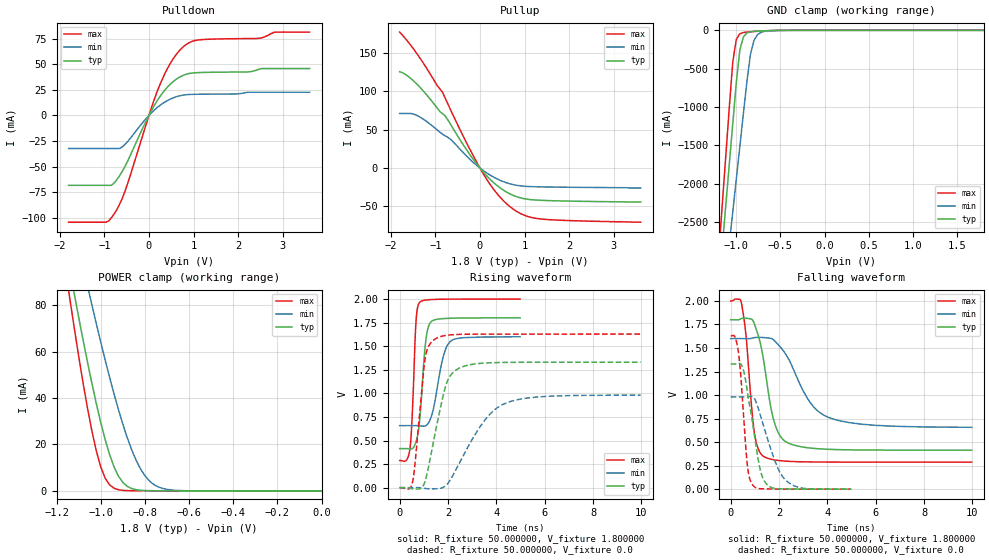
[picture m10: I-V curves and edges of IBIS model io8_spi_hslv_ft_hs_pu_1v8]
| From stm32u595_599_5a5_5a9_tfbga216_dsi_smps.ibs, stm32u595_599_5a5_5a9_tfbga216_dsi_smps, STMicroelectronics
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|   Model io8_spi_hslv_ft_hs_pu_1v8
[Model]  io8_spi_hslv_ft_hs_pu_1v8
Model_type I/O
Polarity   Non-Inverting
Enable   Active-Low
Vinl =   0.540000V
Vinh =   1.260000V
Vmeas =  0.900000V
Cref =   50.000000pF
Rref =   100.000000M
Vref =   0.0V
C_comp   3.338700pF   3.332500pF   3.379000pF
[Temperature Range]   25.000000   0.140000k   -40.000000
[Pullup Reference]   1.800000V   1.600000V   2.000000V
[Pulldown Reference]   0.0V   0.0V   0.0V
[POWER Clamp Reference]   1.800000V   1.600000V   2.000000V
[GND Clamp Reference]   0.0V   0.0V   0.0V
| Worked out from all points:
|   slope of the pulldown table from 0 to 0.27 V, typ, clamps not added: 13.6 ohm
|   slope of the pullup table from 0 to 0.27 V, typ, clamps not added: 15.9 ohm
|   GND clamp passes 1 mA (typ) near -0.51 V on its own axis
|   POWER clamp passes 1 mA (typ) near -0.86 V on its own axis
|   rising waveform, R_fixture 50.000000, V_fixture 1.800000: 20-80 % time 248ps typ, 425ps min, 162ps max; typ from 0.415 V to 1.8 V
|   rising waveform, R_fixture 50.000000, V_fixture 0.0: 20-80 % time 658ps typ, 1.41ns min, 354ps max; typ from 0 V to 1.33 V
|   falling waveform, R_fixture 50.000000, V_fixture 1.800000: 20-80 % time 579ps typ, 1.21ns min, 341ps max; typ from 1.8 V to 0.415 V
|   falling waveform, R_fixture 50.000000, V_fixture 0.0: 20-80 % time 499ps typ, 774ps min, 276ps max; typ from 1.33 V to 0 V
[Pulldown]
|Voltage   I(typ)   I(min)   I(max)
-1.8V     -68.38mA   -32.32mA   -104.4mA
-960mV    -68.38mA   -32.32mA   -104.4mA
-780mV    -66.07mA   -32.32mA   -96.42mA
-540mV    -50.22mA   -28.51mA   -74.66mA
0V        0A         0A         0A
240mV     18.04mA    9.599mA    29.41mA
480mV     30.68mA    16.02mA    50.95mA
780mV     39.47mA    19.98mA    67.56mA
1.14V     41.98mA    20.78mA    74.01mA
2.46V     45.09mA    22.68mA    75.44mA
2.82V     45.89mA    22.68mA    81.56mA
3.6V      45.89mA    22.68mA    81.56mA
[Pullup]
|Voltage   I(typ)   I(min)   I(max)
-1.8V     125.5mA    71.12mA    177.1mA
-1.5V     114.2mA    70.55mA    156mA
-1.32V    103.6mA    65.58mA    141.1mA
-840mV    70.93mA    44.11mA    98.76mA
-660mV    57.08mA    37.46mA    76.03mA
-360mV    29.01mA    19.22mA    39.75mA
60mV      -4.209mA   -2.643mA   -6.075mA
360mV     -21.65mA   -13.44mA   -31.67mA
660mV     -33.29mA   -20.31mA   -49.69mA
960mV     -39.54mA   -23.52mA   -60.64mA
1.32V     -41.88mA   -24.45mA   -66.02mA
3.6V      -44.3mA    -26mA      -70.5mA
[GND_clamp]
|Voltage   I(typ)   I(min)   I(max)
-1.8V     -9.908A    -9.683A    -9.994A
-1.2V     -3.383A    -4.084A    -2.934A
-1.16V    -2.841A    -3.655A    -2.294A
-1.12V    -2.299A    -3.226A    -1.656A
-1.04V    -1.218A    -2.369A    -414.2mA
-1V       -684.7mA   -1.941A    -119.2mA
-960mV    -257.2mA   -1.514A    -45.66mA
-920mV    -87.03mA   -1.089A    -28.93mA
-840mV    -19.35mA   -312.8mA   -18.96mA
-800mV    -13.55mA   -132.4mA   -15.49mA
-720mV    -8.042mA   -25.66mA   -9.49mA
1.8V      0A         13.64nA    0A
[POWER_clamp]
|Voltage   I(typ)   I(min)   I(max)
-1.8V     470.9mA    433.7mA    554.6mA
-1.14V    95.28mA    122.7mA    82.88mA
-1.12V    85mA       114mA      70.34mA
-1.06V    55.55mA    88.43mA    35.73mA
-1.04V    46.38mA    80.17mA    25.83mA
-1V       29.54mA    64.14mA    10.37mA
-940mV    10.43mA    41.88mA    1.177mA
-900mV    3.66mA     28.79mA    250.5uA
-840mV    527.2uA    13.26mA    95.94uA
-800mV    154uA      6.55mA     88.41uA
-740mV    59.83uA    1.741mA    70.38uA
0V        0A         18.18nA    0A
[Ramp]
| variable   typ   min   max
dV/dt_r  0.79756/0.65629n   0.58781/1.41201n   0.97651/0.35346n
dV/dt_f  0.83129/0.57799n   0.56431/1.20386n   1.02742/0.34085n
R_load = 50.000000
[Rising Waveform]
R_fixture= 50.000000
V_fixture= 1.800000
V_fixture_min= 1.600000
V_fixture_max= 2.000000
|time   V(typ)   V(min)   V(max)
0s        414.5mV    657.6mV    287.8mV
440.4ps   408.4mV    657.7mV    442.3mV
530.5ps   414.7mV    657.8mV    823.4mV
670.7ps   480.5mV    657.7mV    1.731V
820.8ps   695.4mV    656mV      1.961V
1.081ns   1.554V     657.1mV    1.988V
1.301ns   1.758V     748.1mV    1.994V
1.802ns   1.792V     1.385V     1.998V
2.082ns   1.795V     1.547V     1.998V
4.985ns   1.8V       1.6V       1.999V
[Rising Waveform]
R_fixture= 50.000000
V_fixture= 0.0
V_fixture_min= 0.0
V_fixture_max= 0.0
|time   V(typ)   V(min)   V(max)
0s        405.1uV    502.6uV    493.5uV
520.5ps   -10.97mV   536.3uV    44.51mV
620.6ps   -13.8mV    627.3uV    214.3mV
1.061ns   74.82mV    -7.697mV   1.383V
1.481ns   593.5mV    -11.54mV   1.578V
1.982ns   1.134V     40.72mV    1.616V
2.683ns   1.289V     363.7mV    1.626V
3.724ns   1.323V     776.7mV    1.628V
4.565ns   1.328V     912.1mV    1.628V
9.97ns    1.33V      980.7mV    1.628V
[Falling Waveform]
R_fixture= 50.000000
V_fixture= 1.800000
V_fixture_min= 1.600000
V_fixture_max= 2.000000
|time   V(typ)   V(min)   V(max)
0s        1.8V       1.6V       1.999V
440.4ps   1.813V     1.6V       1.985V
640.6ps   1.817V     1.599V     1.615V
981ps     1.756V     1.61V      601.7mV
1.361ns   1.371V     1.611V     348.3mV
1.842ns   682.3mV    1.57V      309.9mV
2.422ns   485.8mV    1.37V      295.8mV
3.283ns   437.4mV    923.5mV    289.8mV
4.104ns   423.4mV    757.7mV    288.3mV
9.97ns    414.5mV    657.6mV    287.8mV
[Falling Waveform]
R_fixture= 50.000000
V_fixture= 0.0
V_fixture_min= 0.0
V_fixture_max= 0.0
|time   V(typ)   V(min)   V(max)
0s        1.33V      980.7mV    1.628V
170.2ps   1.33V      980.7mV    1.621V
310.3ps   1.333V     980.8mV    1.474V
510.5ps   1.282V     980.6mV    866.6mV
690.7ps   1.036V     982.1mV    253.9mV
920.9ps   683.2mV    980.6mV    41.17mV
1.171ns   268.9mV    833.8mV    6.215mV
1.361ns   101.8mV    672.3mV    4.108mV
2.262ns   3.374mV    99.5mV     1.132mV
4.985ns   405.1uV    502.6uV    493.5uV
